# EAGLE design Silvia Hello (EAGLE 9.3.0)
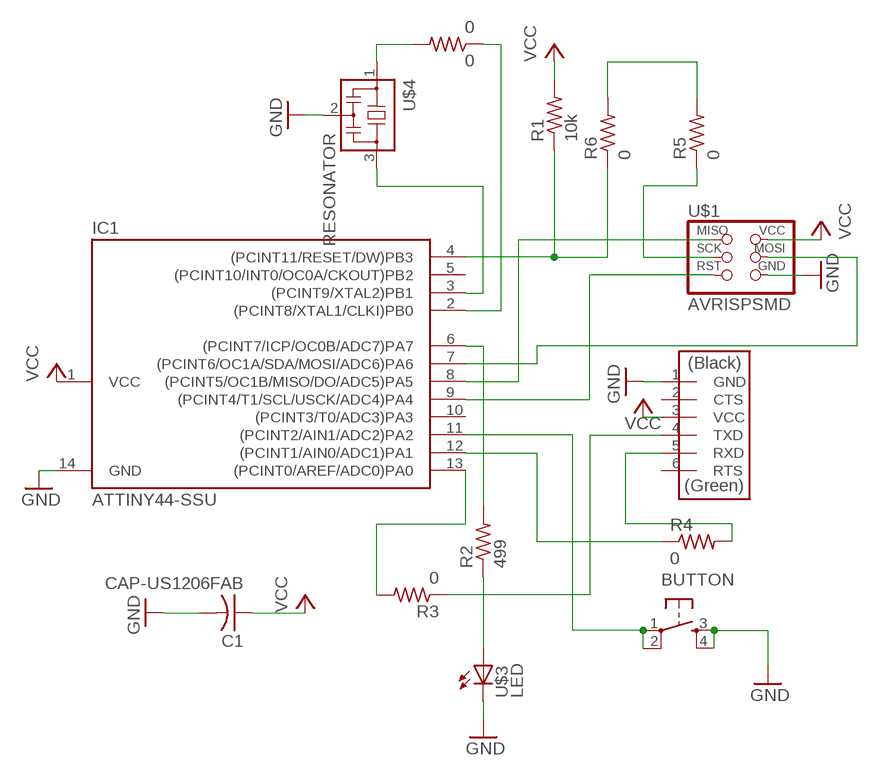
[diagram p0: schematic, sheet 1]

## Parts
0  0  RES-US1206FAB  [R1206FAB]
BUTTON  6MM_SWITCH6MM_SWITCH  [6MM_SWITCH]
C1  CAP-US1206FAB  [C1206FAB]
IC1  ATTINY44-SSU  [SOIC14]
R1  10k  RES-US1206FAB  [R1206FAB]
R2  499  RES-US1206FAB  [R1206FAB]
R3  0  RES-US1206FAB  [R1206FAB]
R4  0  RES-US1206FAB  [R1206FAB]
R5  0  RES-US1206FAB  [R1206FAB]
R6  0  RES-US1206FAB  [R1206FAB]
U$1  AVRISPSMD  [2X03SMD]
U$2  FTDI-SMD-HEADER  [1X06SMD]
U$3  LED  [LED1206]
U$4  RESONATOR  [EFOBM]

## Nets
GND: BUTTON.3(S) BUTTON.4(S1) C1.2 IC1.14(GND) U$1.6(GND) U$2.1(GND) U$3.2(C) U$4.2
N$1: R2.1 U$3.1(A)
N$2: 0.1 IC1.2((PCINT8/XTAL1/CLKI)PB0)
N$3: IC1.3((PCINT9/XTAL2)PB1) U$4.3
N$4: IC1.12((PCINT1/AIN0/ADC1)PA1) R4.1
N$5: R3.1 U$2.4(TXD)
N$6: IC1.6((PCINT7/ICP/OC0B/ADC7)PA7) R2.2
N$7: IC1.9((PCINT4/T1/SCL/USCK/ADC4)PA4) U$1.5(RST)
N$8: BUTTON.1(P) BUTTON.2(P1) IC1.11((PCINT2/AIN1/ADC2)PA2)
N$9: IC1.8((PCINT5/OC1B/MISO/DO/ADC5)PA5) U$1.1(MISO)
N$10: IC1.7((PCINT6/OC1A/SDA/MOSI/ADC6)PA6) U$1.4(MOSI)
N$11: IC1.13((PCINT0/AREF/ADC0)PA0) R3.2
N$12: R4.2 U$2.5(RXD)
N$13: 0.2 U$4.1
N$14: R5.2 R6.2
N$15: R5.1 U$1.3(SCK)
N$19: IC1.4((PCINT11/RESET/DW)PB3) R1.1 R6.1
VCC: C1.1 IC1.1(VCC) R1.2 U$1.2(VCC) U$2.3(VCC)
Unconnected: IC1.5((PCINT10/INT0/OC0A/CKOUT)PB2) IC1.10((PCINT3/T0/ADC3)PA3) U$2.2(CTS) U$2.6(RTS)

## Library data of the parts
0 R1-R6 = fab:RES-US: Resistor (US Symbol)
BUTTON = fab:6MM_SWITCH: OMRON SWITCH
C1 = fab:CAP-US
IC1 = fab:ATTINY44
U$1 = fab:AVRISP
U$2 = fab:FTDI-SMD-HEADER
U$3 = fab:LED: LED
U$4 = fab:RESONATOR

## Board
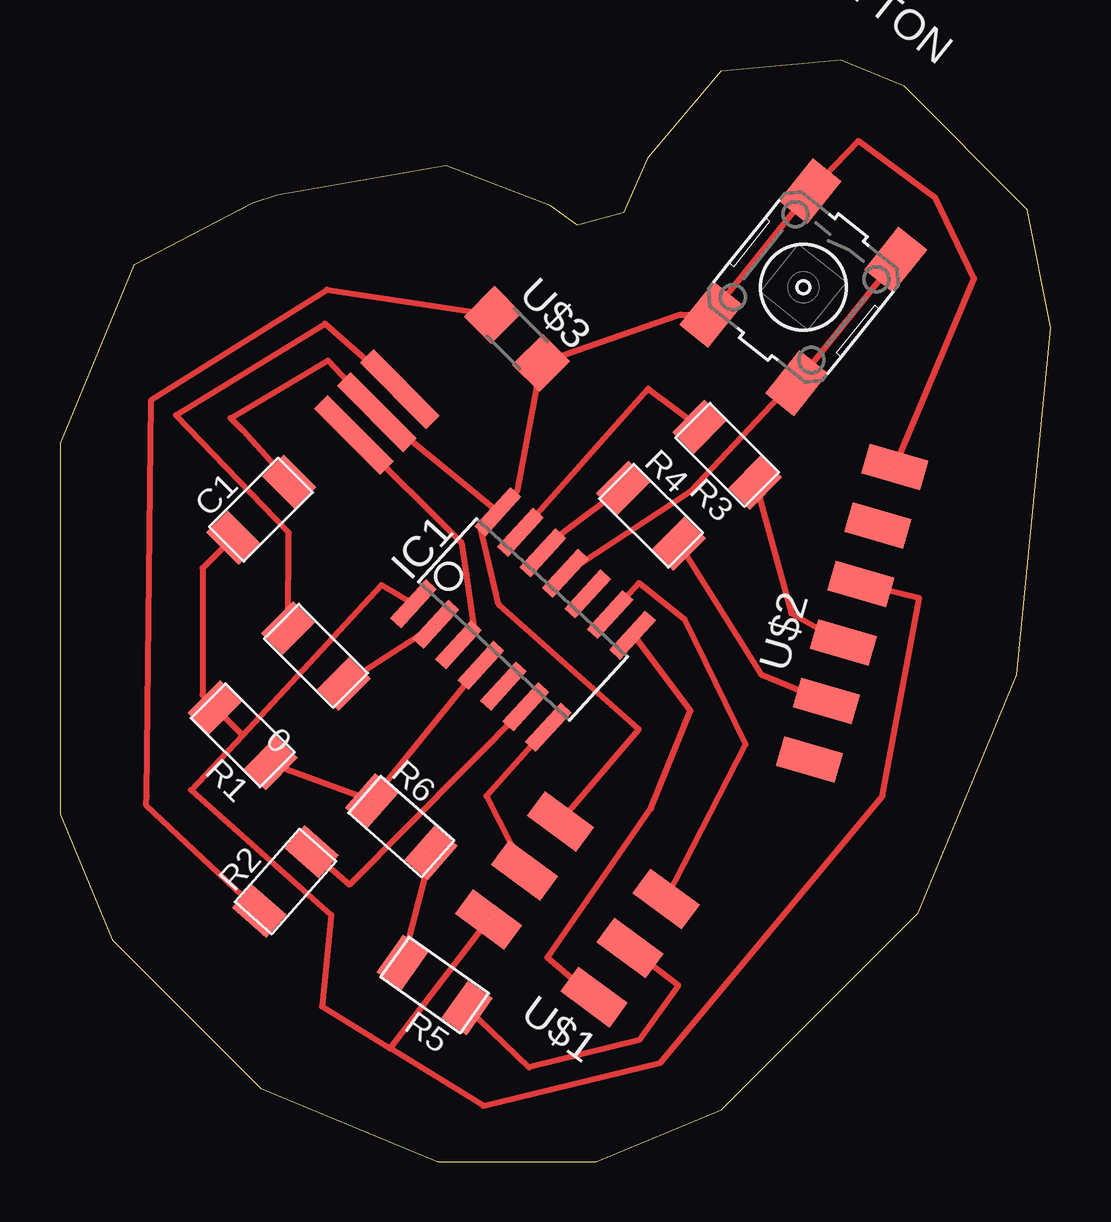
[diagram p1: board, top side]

Size 41.31 x 45.91 mm. Coordinates in mm from the lower left corner, seen from the top.
Outline: 16.1,41.52 20.44,39.84 21.58,39.02 23.49,39.54 24.49,41.82 27.55,45.45 32.55,45.91 35.19,44.82 40.33,39.68 41.31,34.76 39.89,20.3 35.78,10.38 27.57,2.17 22.33,0 15.77,0 8.36,3.07 2.17,9.26 0,14.5 0,29.95 3.07,37.36
Outline: 16.1,41.52 16.1,41.52
Outline: 16.1,41.52 16.1,41.52
Outline: 16.1,41.52 9.05,40.28 8.03,39.94 3.07,37.36
Outline: 3.07,37.36 3.07,37.36
Copper layers (1*16): Top 0.035mm / dielectric 1.5mm / Bottom 0.035mm
Design rules "default": minimum track width 6mil, minimum drill 0.35mm, track to track 6mil, track to pad 6mil, pad to pad 6mil, via to via 6mil, smd to smd 6mil, copper to edge 40mil, drill to drill 6mil, minimum pad ring 10mil, minimum via ring 8mil, stop-mask expansion 4mil, vias tented up to drill 0mil, thermal gap 10mil

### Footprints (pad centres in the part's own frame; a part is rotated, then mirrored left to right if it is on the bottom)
R1206FAB = smd 1.27 x 1.905: 1 -1.651,0; 2 1.651,0
6MM_SWITCH = smd 2.286 x 1.524: 1 -3.302,2.286; 2 3.302,2.286; 3 -3.302,-2.286; 4 3.302,-2.286
C1206FAB = smd 1.27 x 1.905: 1 -1.651,0; 2 1.651,0
SOIC14 = smd 0.61 x 2.21: 1 -3.81,-2.603; 2 -2.54,-2.603; 3 -1.27,-2.603; 4 0,-2.603; 5 1.27,-2.603; 6 2.54,-2.603; 7 3.81,-2.603; 8 3.81,2.603; 9 2.54,2.603; 10 1.27,2.603; 11 0,2.603; 12 -1.27,2.603; 13 -2.54,2.603; 14 -3.81,2.603
2X03SMD = smd 2.54 x 1.27: 1 -2.54,2.54; 2 2.92,2.54; 3 -2.54,0; 4 2.92,0; 5 -2.54,-2.54; 6 2.92,-2.54
1X06SMD = smd 2.54 x 1.27: 1 0,6.35; 2 0,3.81; 3 0,1.27; 4 0,-1.27; 5 0,-3.81; 6 0,-6.35
LED1206 = smd 1.6 x 1.803: 1 -1.422,0; 2 1.422,0
EFOBM = smd 0.8 x 3.9: 1 -1.35,0; 2 0,0; 3 1.35,0

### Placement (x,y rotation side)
0  10.67,21.08 135 top
BUTTON  30.99,36.45 231.3 top
C1  8.38,27.18 45 top
IC1  19.3,22.61 317.5 top
R1  7.62,17.78 135.1 top
R2  9.4,11.68 48.6 top
R3  27.81,29.46 135 top
R4  24.64,26.92 315 top
R5  15.62,7.37 144.8 top
R6  14.22,13.97 318.7 top
U$1  21.72,10.41 143.7 top
U$2  33.02,22.86 343.7 top
U$3  19.05,34.29 315 top
U$4  13.21,31.24 225 top

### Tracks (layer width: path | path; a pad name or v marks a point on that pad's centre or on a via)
GND  (7 unrouted)
  Top 0.152: 17.98,26.82 18.14,26.98 | 18.14,26.98 IC1.14 | IC1.14 | 35.92,28.55 U$2.1 34.8,29.01 | 30.94,40.36 BUTTON.3 | 17.53,26.42 IC1.14 | 11.48,33.07 11.18,33.4 | 19.05,27.94 18.14,26.98
  Top 0.254: IC1.14 U$4.2 11.18,33.4 7.11,30.99 7.62,30.48 C1.2 | 34.8,29.01 38.1,36.83 36.49,40.18 33.27,42.55 BUTTON.3 BUTTON.4 25.87,35.3 U$3.2 19.05,27.94 | U$1.6 24.13,18.03 18.29,23.24 17.53,26.42
N$1  (2 unrouted)
  Top 0.254: R2.1 3.6,14.85 3.62,15.25 3.81,31.75 11.13,36.35 U$3.1
N$2  (2 unrouted)
  Top 0.152: 0.1 12.23,19.91
  Top 0.254: 0.1 IC1.2
N$3  (2 unrouted)
  Top 0.152: 16.61,21.64 IC1.3 | 12.34,30.18 U$4.3
  Top 0.203: IC1.3 17.27,22.23
  Top 0.254: 12.34,30.18 16.75,25.77 17.27,22.23
N$4  (2 unrouted)
  Top 0.254: R4.1 20.99,26.25 IC1.12
N$5  (2 unrouted)
  Top 0.254: R3.1 30.48,22.86 U$2.4
N$6  (2 unrouted)
  Top 0.254: R2.2 12.06,11.56 IC1.6
N$7  (2 unrouted)
  Top 0.152: 22.86,22.71 IC1.9
  Top 0.254: IC1.9 24.13,24.13 26.04,22.61 28.57,17.4 U$1.5
N$8  (3 unrouted)
  Top 0.152: 21.18,24.54 IC1.11 | BUTTON.2 30.11,31.85 29.97,31.88
  Top 0.254: BUTTON.1 BUTTON.2 | IC1.11 26.29,27.94 29.97,31.88
N$9  (2 unrouted)
  Top 0.152: 23.93,21.95 IC1.8
  Top 0.254: U$1.1 20.32,8.51 24.64,14.73 26.29,18.8 23.93,21.95
N$10  (2 unrouted)
  Top 0.152: 20.42,17.98 IC1.7
  Top 0.254: IC1.7 17.78,15.24 U$1.4
N$11  (2 unrouted)
  Top 0.254: IC1.13 24.51,32.23 R3.2
N$12  (2 unrouted)
  Top 0.254: R4.2 29.21,20.32 U$2.5
N$13  (2 unrouted)
  Top 0.254: U$4.1 11.05,34.92 4.83,31.11 9.54,26.21 0.2
N$14  (2 unrouted)
  Top 0.254: R6.2 R5.2
N$15  (2 unrouted)
  Top 0.254: U$1.3 25.78,7.37 24.13,5.08 19.56,3.94 R5.1
N$19  (3 unrouted)
  Top 0.152: 18.14,21.18 17.68,20.73 IC1.4
  Top 0.254: R1.1 R6.1 IC1.4
VCC  (5 unrouted)
  Top 0.152: 6.5,18.85 R1.2 | 33.63,23.98 33.42,24.06 U$2.3
  Top 0.254: C1.1 5.95,24.74 5.94,19.45 R1.2 7.62,17.78 | 7.62,17.78 13.4,24.04 IC1.1 | 33.42,24.06 35.81,23.5 34.29,15.24 25.02,4.12 17.65,2.33 13.76,4.73 | 7.62,17.78 5.46,15.49 11.3,10.29 10.92,6.48 13.76,4.73 | U$1.2 13.76,4.73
